(* Logix 5000 AddOnInstructionDefinition export Banner_K50Z_Param_v4; software revision 33.00; part 3 of 3 *)
(* tags used below, declared in another part *)
   K50Z : Banner_K50Z_v4;
   Port_Data : Banner_IOL_Port_v4;
   Port : DINT;
   Local_Control : DINT;
   Command_Being_Processed : BOOL;
   Update_Archive : BOOL;
   Index_Write_Inprocess : INT;
   Inprocess_Index : DINT;
(* Banner_K50Z_Param_v4, continued *)

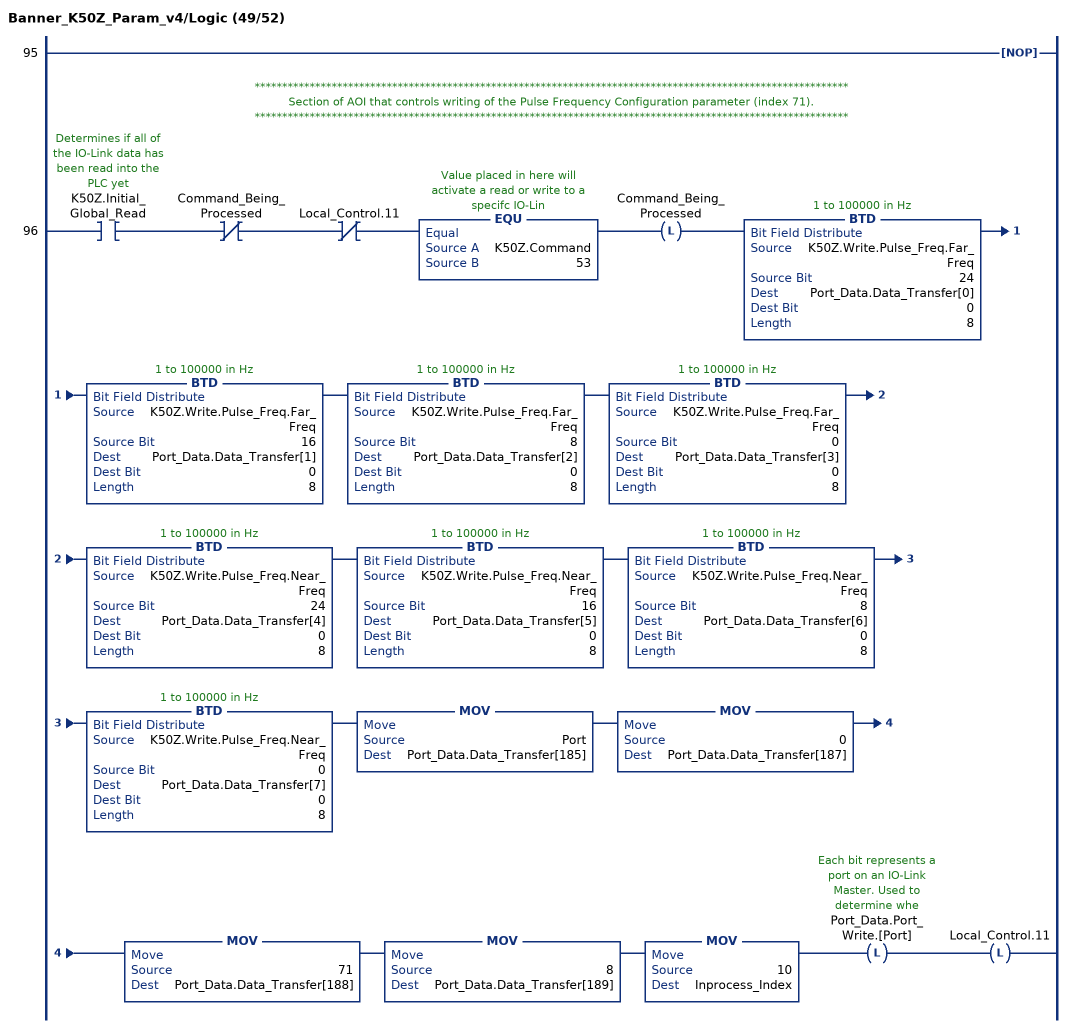
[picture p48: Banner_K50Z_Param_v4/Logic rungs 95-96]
   95: NOP();
   // ************************************************************************************************************
   // Section of AOI that controls writing of the Pulse Frequency Configuration parameter (index 71).
   // ************************************************************************************************************
   96: XIC(K50Z.Initial_Global_Read)XIO(Command_Being_Processed)XIO(Local_Control.11)EQU(K50Z.Command,53)OTL(Command_Being_Processed)BTD(K50Z.Write.Pulse_Freq.Far_Freq,24,Port_Data.Data_Transfer[0],0,8)BTD(K50Z.Write.Pulse_Freq.Far_Freq,16,Port_Data.Data_Transfer[1],0,8)BTD(K50Z.Write.Pulse_Freq.Far_Freq,8,Port_Data.Data_Transfer[2],0,8)BTD(K50Z.Write.Pulse_Freq.Far_Freq,0,Port_Data.Data_Transfer[3],0,8)BTD(K50Z.Write.Pulse_Freq.Near_Freq,24,Port_Data.Data_Transfer[4],0,8)BTD(K50Z.Write.Pulse_Freq.Near_Freq,16,Port_Data.Data_Transfer[5],0,8)BTD(K50Z.Write.Pulse_Freq.Near_Freq,8,Port_Data.Data_Transfer[6],0,8)BTD(K50Z.Write.Pulse_Freq.Near_Freq,0,Port_Data.Data_Transfer[7],0,8)MOV(Port,Port_Data.Data_Transfer[185])MOV(0,Port_Data.Data_Transfer[187])MOV(71,Port_Data.Data_Transfer[188])MOV(8,Port_Data.Data_Transfer[189])MOV(10,Inprocess_Index)OTL(Port_Data.Port_Write.[Port])OTL(Local_Control.11);
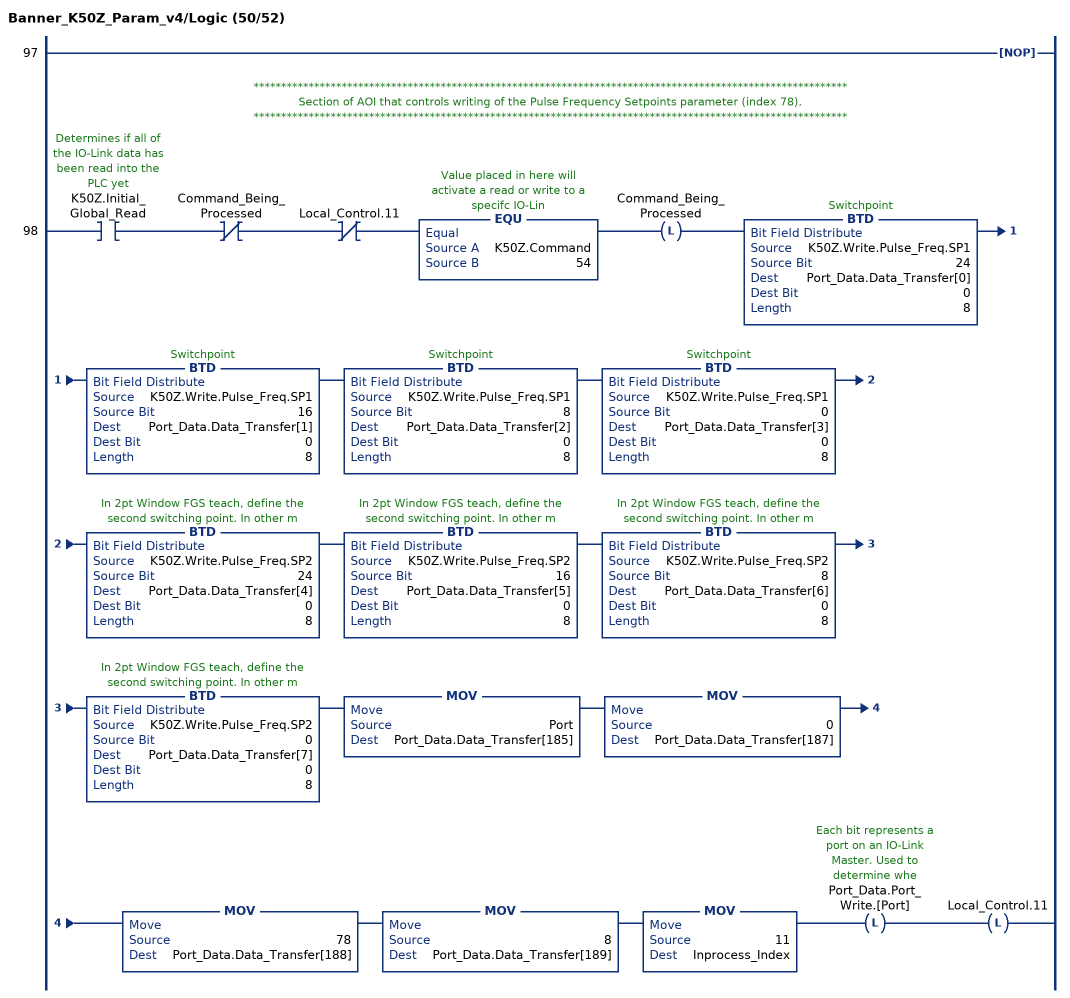
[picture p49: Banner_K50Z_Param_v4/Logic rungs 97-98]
   97: NOP();
   // ************************************************************************************************************
   // Section of AOI that controls writing of the Pulse Frequency Setpoints parameter (index 78).
   // ************************************************************************************************************
   98: XIC(K50Z.Initial_Global_Read)XIO(Command_Being_Processed)XIO(Local_Control.11)EQU(K50Z.Command,54)OTL(Command_Being_Processed)BTD(K50Z.Write.Pulse_Freq.SP1,24,Port_Data.Data_Transfer[0],0,8)BTD(K50Z.Write.Pulse_Freq.SP1,16,Port_Data.Data_Transfer[1],0,8)BTD(K50Z.Write.Pulse_Freq.SP1,8,Port_Data.Data_Transfer[2],0,8)BTD(K50Z.Write.Pulse_Freq.SP1,0,Port_Data.Data_Transfer[3],0,8)BTD(K50Z.Write.Pulse_Freq.SP2,24,Port_Data.Data_Transfer[4],0,8)BTD(K50Z.Write.Pulse_Freq.SP2,16,Port_Data.Data_Transfer[5],0,8)BTD(K50Z.Write.Pulse_Freq.SP2,8,Port_Data.Data_Transfer[6],0,8)BTD(K50Z.Write.Pulse_Freq.SP2,0,Port_Data.Data_Transfer[7],0,8)MOV(Port,Port_Data.Data_Transfer[185])MOV(0,Port_Data.Data_Transfer[187])MOV(78,Port_Data.Data_Transfer[188])MOV(8,Port_Data.Data_Transfer[189])MOV(11,Inprocess_Index)OTL(Port_Data.Port_Write.[Port])OTL(Local_Control.11);
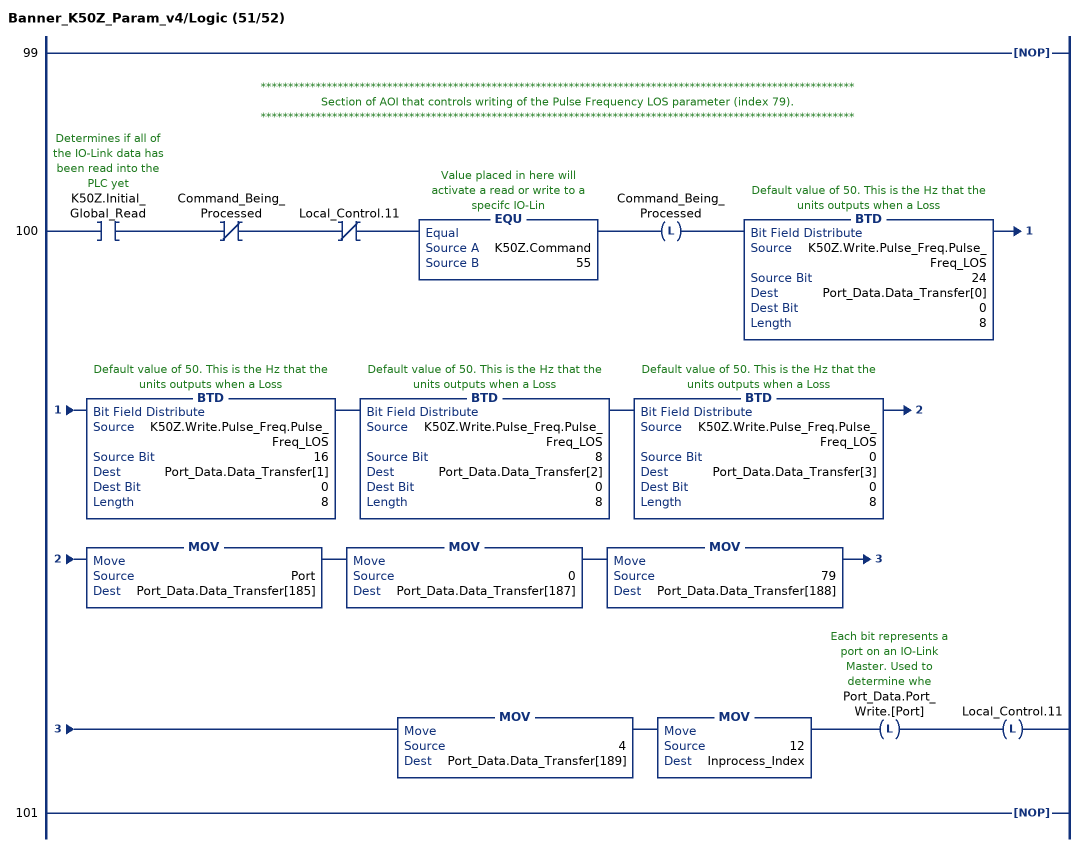
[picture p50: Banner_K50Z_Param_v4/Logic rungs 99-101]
   99: NOP();
   // ************************************************************************************************************
   // Section of AOI that controls writing of the Pulse Frequency LOS parameter (index 79).
   // ************************************************************************************************************
   100: XIC(K50Z.Initial_Global_Read)XIO(Command_Being_Processed)XIO(Local_Control.11)EQU(K50Z.Command,55)OTL(Command_Being_Processed)BTD(K50Z.Write.Pulse_Freq.Pulse_Freq_LOS,24,Port_Data.Data_Transfer[0],0,8)BTD(K50Z.Write.Pulse_Freq.Pulse_Freq_LOS,16,Port_Data.Data_Transfer[1],0,8)BTD(K50Z.Write.Pulse_Freq.Pulse_Freq_LOS,8,Port_Data.Data_Transfer[2],0,8)BTD(K50Z.Write.Pulse_Freq.Pulse_Freq_LOS,0,Port_Data.Data_Transfer[3],0,8)MOV(Port,Port_Data.Data_Transfer[185])MOV(0,Port_Data.Data_Transfer[187])MOV(79,Port_Data.Data_Transfer[188])MOV(4,Port_Data.Data_Transfer[189])MOV(12,Inprocess_Index)OTL(Port_Data.Port_Write.[Port])OTL(Local_Control.11);
   101: NOP();
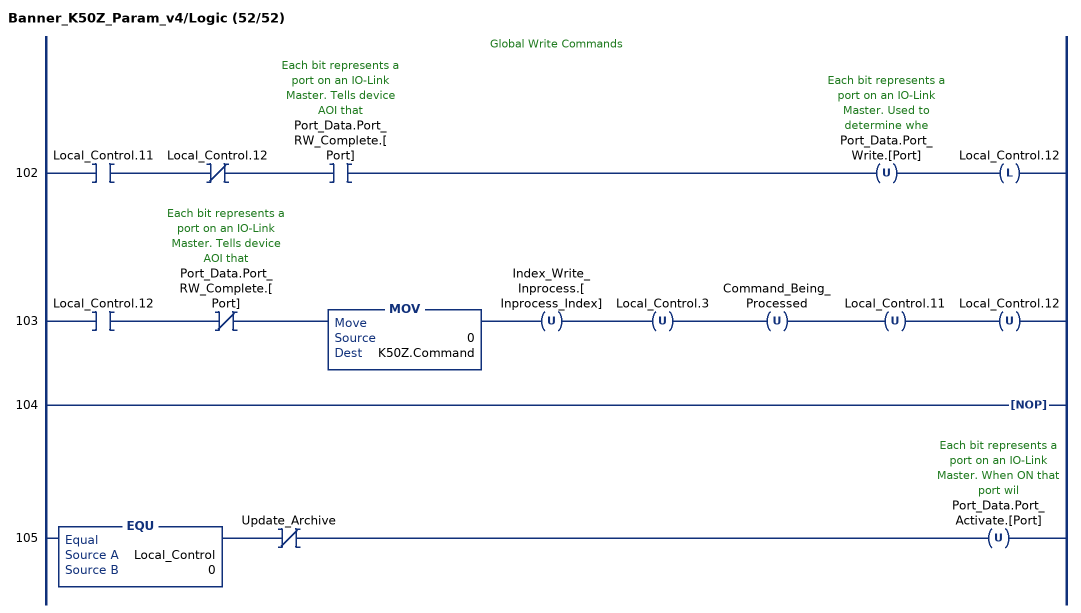
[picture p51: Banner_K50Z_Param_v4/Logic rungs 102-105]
   // Global Write Commands
   102: XIC(Local_Control.11)XIO(Local_Control.12)XIC(Port_Data.Port_RW_Complete.[Port])OTU(Port_Data.Port_Write.[Port])OTL(Local_Control.12);
   103: XIC(Local_Control.12)XIO(Port_Data.Port_RW_Complete.[Port])MOV(0,K50Z.Command)OTU(Index_Write_Inprocess.[Inprocess_Index])OTU(Local_Control.3)OTU(Command_Being_Processed)OTU(Local_Control.11)OTU(Local_Control.12);
   104: NOP();
   105: EQU(Local_Control,0)XIO(Update_Archive)OTU(Port_Data.Port_Activate.[Port]);
END_ROUTINE
END_ADD_ON_INSTRUCTION
